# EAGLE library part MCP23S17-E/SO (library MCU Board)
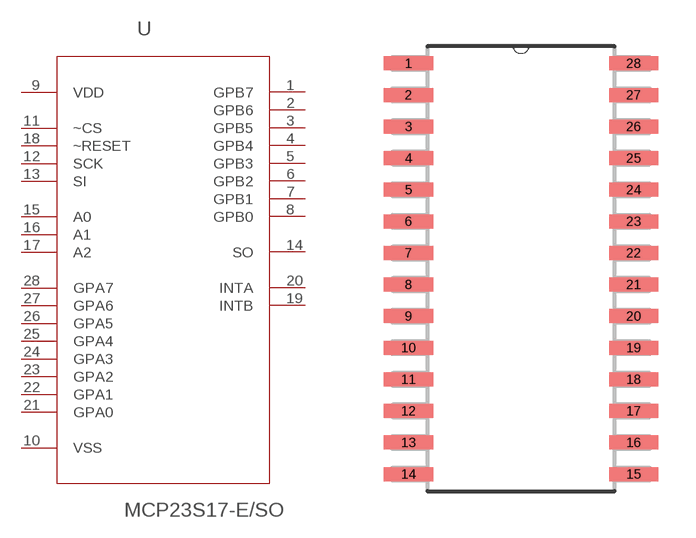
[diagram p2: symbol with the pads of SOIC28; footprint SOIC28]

Designator prefix U

## MCP23S17-E/SO  [SOIC28]
1  GPB7
2  GPB6
3  GPB5
4  GPB4
5  GPB3
6  GPB2
7  GPB1
8  GPB0
9  VDD  pwr
10  VSS  pwr
11  ~CS  in
12  SCK  in
13  SI  in
14  SO  out
15  A0  in
16  A1  in
17  A2  in
18  ~RESET  in
19  INTB  out
20  INTA  out
21  GPA0
22  GPA1
23  GPA2
24  GPA3
25  GPA4
26  GPA5
27  GPA6
28  GPA7

## Footprint SOIC28 (pad centres in mm)
smd 1.981 x 0.559: 1 -4.521,8.255; 2 -4.521,6.985; 3 -4.521,5.715; 4 -4.521,4.445; 5 -4.521,3.175; 6 -4.521,1.905; 7 -4.521,0.635; 8 -4.521,-0.635; 9 -4.521,-1.905; 10 -4.521,-3.175; 11 -4.521,-4.445; 12 -4.521,-5.715; 13 -4.521,-6.985; 14 -4.521,-8.255; 15 4.521,-8.255; 16 4.521,-6.985; 17 4.521,-5.715; 18 4.521,-4.445; 19 4.521,-3.175; 20 4.521,-1.905; 21 4.521,-0.635; 22 4.521,0.635; 23 4.521,1.905; 24 4.521,3.175; 25 4.521,4.445; 26 4.521,5.715; 27 4.521,6.985; 28 4.521,8.255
